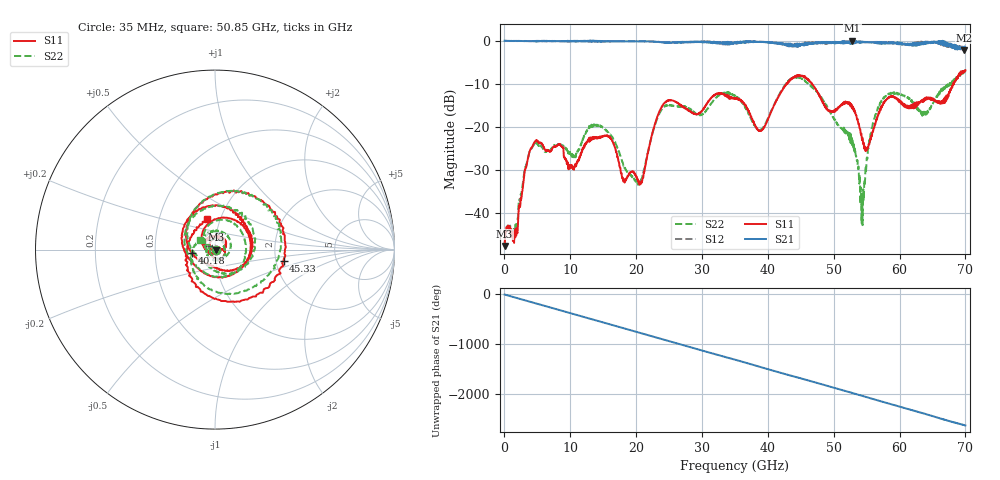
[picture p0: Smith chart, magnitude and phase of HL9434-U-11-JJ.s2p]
! 7/27/2020 1:01:21 PM
! H:\PRODUCTION_DATA\TEMP_S2P.S2P
! CHANNEL.1
! TR.MEASUREMENT
! CORRECTED.DATA
# GHZ S RI R 50.0
! FREQ.GHZ  S11RE  S11IM  S21RE  S21IM  S12RE  S12IM  S22RE  S22IM
!; PortSelection: Port_12
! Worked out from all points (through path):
!   2000 points, 35 MHz to 70 GHz, reference 50 ohm
!   highest |S21| = 0.02 dB at 52.85 GHz (marker M1); lowest = -2.2 dB at 69.79 GHz (marker M2)
!   group delay of S21, straight-line fit = 104 ps
!   lowest |S11| = -47.5 dB at 35 MHz (marker M3), VSWR 1.01, Z = 50.4 - j0.0322 ohm
!   |S11| at or under -10 dB: start of sweep to 42.84 GHz; 42.85044 GHz to 42.8789 GHz (28.46 MHz wide, 0.0664 % of centre); 46.72 GHz to 68.13 GHz (21.41 GHz wide, 37.3 % of centre)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
!   |S22| runs from -47.6 to -6.9 dB; largest |S21 - S12| = 0.12
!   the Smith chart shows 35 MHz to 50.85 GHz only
!   S11 on the Smith chart (normalised r, x): 35 MHz: 1.01, -0.00; 40.18 GHz: 0.77, -0.03; 45.33 GHz: 2.21, -0.32; 50.85 GHz: 0.87, +0.30
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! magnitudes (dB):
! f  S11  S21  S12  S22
! 35 MHz  -47.5  0.0  0.0  -47.6
! 1.75 GHz  -43.8  -0.1  -0.1  -43.0
! 3.325 GHz  -29.2  -0.1  -0.1  -28.9
! 4.62 GHz  -23.5  -0.1  -0.1  -23.9
! 10.22 GHz  -29.2  -0.2  -0.1  -26.9
! 11.72 GHz  -25.7  -0.1  -0.1  -23.7
! 14.84 GHz  -22.2  -0.2  -0.2  -19.9
! 20.41 GHz  -32.5  -0.2  -0.2  -33.1
! 23.38 GHz  -17.0  -0.3  -0.3  -17.4
! 35.03 GHz  -13.3  -0.5  -0.5  -12.7
! 38.53 GHz  -20.8  -0.2  -0.3  -20.7
! 40.18 GHz  -17.7  -0.4  -0.4  -17.4
! 45.33 GHz  -8.2  -0.8  -0.7  -9.0
! 46.69 GHz  -9.9  -0.7  -0.5  -10.7
! 50.85 GHz  -15.2  -0.4  -0.4  -19.9
! 52.85 GHz  -15.1  0.0  -0.4  -22.7
! 54.39 GHz  -22.5  -0.3  -0.3  -42.7
! 56.07 GHz  -20.2  -0.4  -0.4  -18.8
! 58.34 GHz  -13.1  -0.6  -0.4  -12.3
! 63.8 GHz  -13.8  -0.8  -0.4  -17.4
! 69.79 GHz  -7.2  -2.2  -1.6  -7.0
! 70 GHz  -6.9  -1.7  -1.8  -7.2
